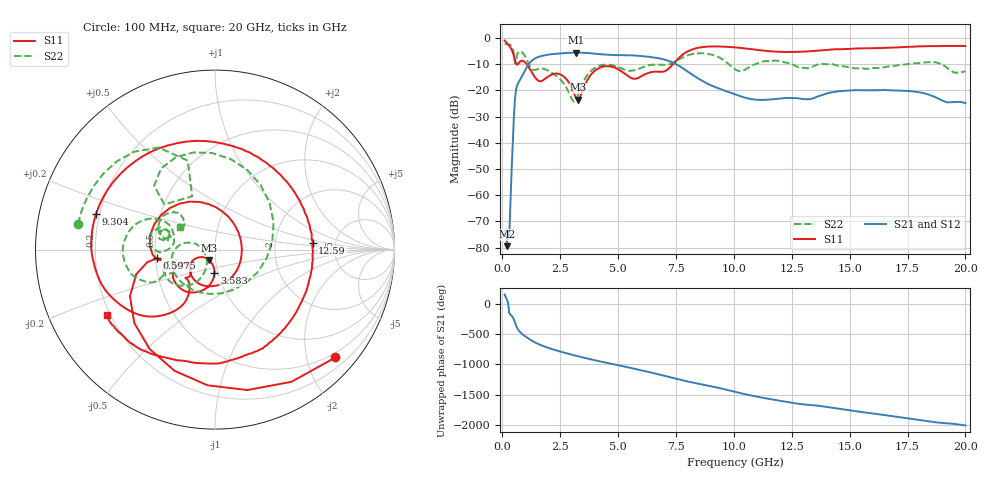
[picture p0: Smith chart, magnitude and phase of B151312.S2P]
!  2-Port S-parameters saved by WinCal
! VAR MeasName=S-Parameters (CALIBRATED_DATA) read from VNA (N5244A)
! VAR MeasDate=12/8/2015 5:43:23 PM
! VAR NAME=B151312
! VAR FILENAME=B151312.S2P
! VAR DATE=12/8/2015 5:43:23 PM
! VAR PHYS_PORTS=1,2
# Hz S DB R 50
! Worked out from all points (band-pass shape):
!   401 points, 100 MHz to 20 GHz, reference 50 ohm
!   highest |S21| = -5.54 dB at 3.184 GHz (marker M1); lowest = -79.5 dB at 199.5 MHz (marker M2)
!   |S21| within 3 dB of the highest: 1.288 GHz to 7.127 GHz (5.839 GHz wide, 139 % of centre)
!   lowest |S11| = -23.5 dB at 3.284 GHz (marker M3), VSWR 1.14, Z = 46.4 - j5.34 ohm
!   |S11| at or under -10 dB: 624.1 MHz to 673.2 MHz (49.14 MHz wide, 7.58 % of centre); 1.061 GHz to 7.367 GHz (6.307 GHz wide, 150 % of centre)
!   |S22| runs from -24.3 to -2.2 dB; largest |S21 - S12| = 0.0021
!   S11 on the Smith chart (normalised r, x): 100 MHz: 0.40, -2.56; 597.5 MHz: 0.51, -0.06; 3.583 GHz: 0.96, -0.26; 9.304 GHz: 0.19, +0.14; 12.59 GHz: 3.36, +0.38; 20 GHz: 0.19, -0.27
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1e8  -0.91 -41.8  -75.54 155.0  -79.77 140.9  -2.19 169.3
1.995e8  -1.91 -77.0  -79.49 73.0  -81.39 85.7  -2.28 158.2
2.99e8  -2.95 -108.5  -76.28 -148.0  -81.71 -92.9  -2.48 145.5
5.975e8  -9.72 -171.4  -19.42 -0.6  -19.41 -0.6  -8.45 138.3
1.095e9  -10.41 117.6  -10.56 156.1  -10.56 156.1  -8.87 25.0
1.493e9  -15.85 35.5  -7.44 68.1  -7.44 68.2  -11.94 -109.0
2.04025e9  -14.38 -73.9  -6.26 -14.4  -6.26 -14.3  -12.72 -176.7
3.1845e9  -22.88 -141.1  -5.54 -137.5  -5.54 -137.5  -23.62 -135.7
3.284e9  -23.50 -121.0  -5.54 -147.1  -5.54 -147.1  -21.43 -121.8
3.43325e9  -20.91 -96.5  -5.58 -161.3  -5.57 -161.3  -17.96 -115.6
3.5825e9  -17.66 -91.4  -5.65 -175.2  -5.64 -175.2  -15.32 -116.2
4.82625e9  -11.17 -148.0  -6.48 80.4  -6.47 80.3  -10.55 -161.3
5.7715e9  -15.54 -143.2  -6.68 1.7  -6.68 1.7  -12.16 -153.8
6.7665e9  -12.85 -135.0  -7.72 -86.5  -7.73 -86.6  -10.14 -158.7
8.01025e9  -5.07 -139.4  -12.78 156.2  -12.77 156.1  -6.55 -160.9
9.30375e9  -3.20 163.1  -19.09 53.6  -19.12 53.5  -7.10 159.0
1.005e10  -3.57 132.1  -21.51 -14.8  -21.55 -15.0  -11.90 157.2
1.1244e10  -4.73 75.3  -23.62 -112.3  -23.69 -112.3  -8.97 177.3
1.258725e10  -5.26 4.1  -22.90 159.5  -22.90 160.0  -10.24 158.1
1.338325e10  -4.98 -31.9  -23.15 125.0  -23.09 125.4  -11.06 170.1
1.67165e10  -3.69 -111.1  -19.92 -50.0  -19.74 -50.1  -10.86 168.2
2e10  -3.05 -148.8  -24.86 149.2  -24.87 148.0  -12.73 147.5
